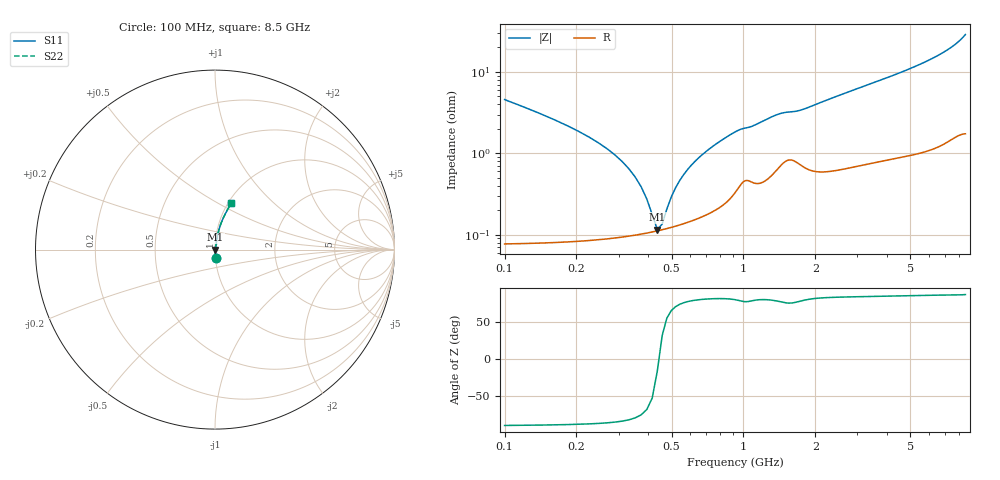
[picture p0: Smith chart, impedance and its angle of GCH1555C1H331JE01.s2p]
!Murata Part Number: GCH1555C1H331JE01
!These Parameters are Measured in Series Mode Connection
!Data Generated on Jun 19, 2026
!  o--ll--o
!Port1  Port2
!  o------o
!Operation Temp=25[degC], DC Bias Voltage=0[V]
!Freq. Start=100[MHz] Stop=9[GHz] 401[Steps]
# Hz S RI R 50
!Freq.(Hz) S11(Real) S11(Imag) S21(Real) S21(Imag) S12(Real) S12(Imag) S22(Real) S22(Imag)
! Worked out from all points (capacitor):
!   401 points, 100 MHz to 8.5 GHz, reference 50 ohm
!   read as one part in series: C = 330 pF near 142 MHz
!   lowest |Z| = 116 mohm at 436 MHz (marker M1)
!   series resonance near 442.5 MHz, so ESL is about 390 pH
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1e8  0.00285 -0.0456  0.9971 0.0456  0.9971 0.0456  0.00285 -0.0456
1.42e8  0.00171 -0.0304  0.9983 0.0304  0.9983 0.0304  0.00171 -0.0304
3.1e8  0.000995 -0.00791  0.999 0.00791  0.999 0.00791  0.000995 -0.00791
3.52e8  0.00101 -0.00502  0.999 0.00502  0.999 0.00502  0.00101 -0.00502
4.15e8  0.00108 -0.00139  0.9989 0.00139  0.9989 0.00139  0.00108 -0.00139
4.36e8  0.00111 -0.000316  0.9989 0.000316  0.9989 0.000316  0.00111 -0.000316
4.57e8  0.00115 0.00071  0.9989 -0.00071  0.9989 -0.00071  0.00115 0.00071
4.78e8  0.00119 0.00169  0.9988 -0.00169  0.9988 -0.00169  0.00119 0.00169
5.41e8  0.00134 0.00443  0.9987 -0.00443  0.9987 -0.00443  0.00134 0.00443
5.83e8  0.00145 0.00612  0.9985 -0.00612  0.9985 -0.00612  0.00145 0.00612
6.67e8  0.00173 0.00927  0.9983 -0.00927  0.9983 -0.00927  0.00173 0.00927
7.72e8  0.0022 0.013  0.9978 -0.013  0.9978 -0.013  0.0022 0.013
9.61e8  0.00424 0.0189  0.9958 -0.0189  0.9958 -0.0189  0.00424 0.0189
1.339e9  0.00642 0.0279  0.9936 -0.0279  0.9936 -0.0279  0.00642 0.0279
1.507e9  0.00889 0.0304  0.9911 -0.0304  0.9911 -0.0304  0.00889 0.0304
1.717e9  0.00833 0.0323  0.9917 -0.0323  0.9917 -0.0323  0.00833 0.0323
2.305e9  0.00807 0.0458  0.9919 -0.0458  0.9919 -0.0458  0.00807 0.0458
2.914e9  0.0103 0.0591  0.9897 -0.0591  0.9897 -0.0591  0.0103 0.0591
4.3e9  0.0167 0.0897  0.9833 -0.0897  0.9833 -0.0897  0.0167 0.0897
5.707e9  0.0265 0.1258  0.9735 -0.1258  0.9735 -0.1258  0.0265 0.1258
7.114e9  0.0452 0.1741  0.9548 -0.1741  0.9548 -0.1741  0.0452 0.1741
8.5e9  0.0903 0.258  0.9097 -0.258  0.9097 -0.258  0.0903 0.258
